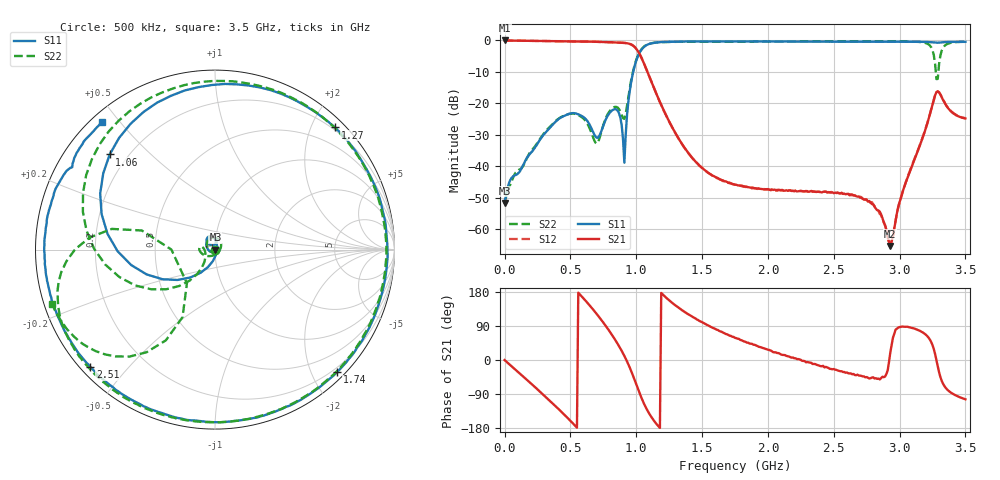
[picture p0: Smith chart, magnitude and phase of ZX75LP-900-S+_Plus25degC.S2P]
! Mini-Circuits
! S2P DATA File Format
! Type:LOW PASS FILTER
! Model: ZX75LP-900-S+
! All S Parameters are in dB deg format
! TEST CONDITIONS: INPUT POWER = 0 dBm @ Temperature = 25 deg C
! 401 Frequency points
# MHz S DB R 50
!FREQ	S11	S11_P	S21	S21_P	S12	S12_P	S22	S22_P
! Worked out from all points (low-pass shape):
!   401 points, 500 kHz to 3.5 GHz, reference 50 ohm
!   highest |S21| = -0.02 dB at 500 kHz (marker M1); lowest = -65.3 dB at 2.93 GHz (marker M2)
!   |S21| within 3 dB of the highest: start of sweep to 1.006 GHz
!   lowest |S11| = -51.7 dB at 1 MHz (marker M3), VSWR 1.01, Z = 50.3 + j0.0254 ohm
!   |S11| at or under -10 dB: start of sweep to 977.3 MHz
!   |S22| runs from -51.8 to -0.3 dB; largest |S21 - S12| = 0.0034
!   S11 on the Smith chart (normalised r, x): 500 kHz: 1.01, +0.00; 1.06 GHz: 0.13, +0.38; 1.27 GHz: 0.16, +2.37; 1.74 GHz: 0.12, -2.40; 2.51 GHz: 0.03, -0.40; 3.5 GHz: 0.03, +0.45
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0.5  -51.43 10.0  -0.02 -0.2  -0.02 -0.2  -51.48 8.6
1  -51.69 5.6  -0.02 -0.3  -0.02 -0.3  -51.75 6.0
300  -29.83 -166.3  -0.20 -93.2  -0.19 -93.2  -29.48 -171.6
590  -24.12 89.4  -0.37 166.4  -0.37 166.3  -24.53 67.7
700  -30.92 102.0  -0.44 121.5  -0.44 121.5  -32.80 -46.3
770  -25.01 138.5  -0.53 89.4  -0.53 89.4  -24.61 -143.9
910  -38.85 -5.6  -0.81 10.7  -0.79 10.7  -24.92 -160.6
990  -7.85 -160.0  -2.18 -54.6  -2.16 -54.7  -7.57 -148.1
1060  -2.04 137.9  -7.42 -115.9  -7.41 -116.1  -1.94 156.8
1170  -0.60 78.3  -18.62 -175.4  -18.66 -175.6  -0.61 100.6
1270  -0.41 45.5  -27.35 151.7  -27.42 151.7  -0.47 69.7
1740  -0.32 -45.1  -45.71 60.9  -45.79 60.7  -0.40 -13.3
1760  -0.33 -47.8  -45.87 57.7  -45.88 58.3  -0.39 -15.9
2340  -0.38 -119.0  -47.98 -10.6  -48.12 -8.4  -0.34 -79.2
2510  -0.41 -136.7  -48.37 -25.5  -48.35 -24.4  -0.33 -94.8
2800  -0.44 -165.7  -52.10 -45.8  -52.06 -46.7  -0.30 -120.1
2920  -0.44 -177.1  -64.04 -4.9  -65.20 -7.5  -0.30 -130.6
2930  -0.45 -178.0  -65.32 20.3  -65.38 14.1  -0.32 -131.5
3210  -0.50 156.2  -26.51 63.2  -26.37 63.8  -1.02 -168.4
3280  -0.72 150.2  -16.47 -0.1  -16.45 1.0  -12.29 179.9
3340  -0.56 146.0  -19.67 -68.4  -19.63 -67.2  -1.81 -132.8
3500  -0.46 131.6  -24.81 -103.7  -24.69 -102.7  -0.39 -161.4
